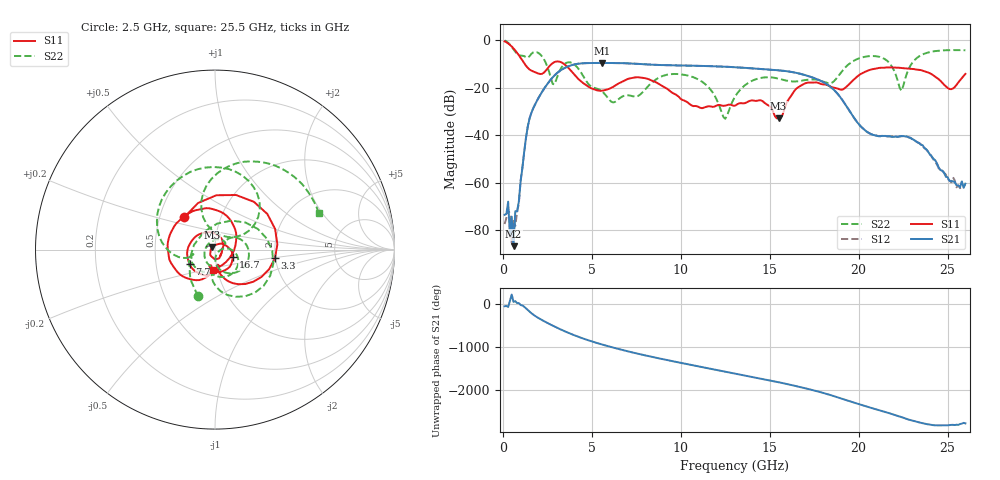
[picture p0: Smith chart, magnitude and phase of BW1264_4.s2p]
!Keysight Technologies,N5245B,MY57181159,A.13.60.06
!Date: Friday, December 18, 2020 23:52:07
!Correction: S11(Full 2 Port(1,2))
!S21(Full 2 Port(1,2))
!S12(Full 2 Port(1,2))
!S22(Full 2 Port(1,2))
!S2P File: Measurements: S11, S21, S12, S22:
# Hz S  dB  R 50
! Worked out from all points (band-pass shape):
!   260 points, 100 MHz to 26 GHz, reference 50 ohm
!   highest |S21| = -9.65 dB at 5.6 GHz (marker M1); lowest = -86.7 dB at 600 MHz (marker M2)
!   |S21| within 3 dB of the highest: 3.273 GHz to 15.35 GHz (12.08 GHz wide, 130 % of centre)
!   lowest |S11| = -33.0 dB at 15.5 GHz (marker M3), VSWR 1.05, Z = 48.3 + j1.35 ohm
!   |S11| at or under -10 dB: 1.223 GHz to 2.759 GHz (1.535 GHz wide, 77.1 % of centre); 3.421 GHz to end of sweep
!   |S22| runs from -33.1 to -0.2 dB; largest |S21 - S12| = 0.00052
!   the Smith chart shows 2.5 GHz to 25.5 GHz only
!   S11 on the Smith chart (normalised r, x): 2.5 GHz: 0.67, +0.26; 3.3 GHz: 1.99, -0.22; 7.7 GHz: 0.74, -0.13; 16.7 GHz: 1.22, -0.10; 25.5 GHz: 0.95, -0.22
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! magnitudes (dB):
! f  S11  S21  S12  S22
! 100 MHz  -0.6  -73.5  -77.4  -0.2
! 300 MHz  -1.5  -68.0  -71.5  -1.2
! 400 MHz  -2.1  -82.7  -73.0  -1.9
! 600 MHz  -3.5  -86.7  -75.3  -3.9
! 1.5 GHz  -12.4  -33.1  -33.0  -6.8
! 2.5 GHz  -12.1  -18.5  -18.5  -11.2
! 3.3 GHz  -9.4  -12.5  -12.5  -11.5
! 4.5 GHz  -18.0  -9.8  -9.8  -14.9
! 5.6 GHz  -21.3  -9.6  -9.6  -21.7
! 7.7 GHz  -15.7  -10.1  -10.1  -23.1
! 8.8 GHz  -18.6  -10.5  -10.5  -15.7
! 11.2 GHz  -28.7  -10.9  -10.9  -17.6
! 12.5 GHz  -27.6  -11.2  -11.2  -33.1
! 13.1 GHz  -27.4  -11.5  -11.5  -23.2
! 15.5 GHz  -33.0  -12.7  -12.7  -16.3
! 16.7 GHz  -19.4  -14.2  -14.2  -17.2
! 17.4 GHz  -17.9  -15.7  -15.7  -16.6
! 21.7 GHz  -11.5  -40.4  -40.6  -9.5
! 22.4 GHz  -11.8  -40.4  -40.5  -21.3
! 23.3 GHz  -12.5  -43.0  -43.0  -7.4
! 25.5 GHz  -18.9  -61.1  -62.0  -4.3
! 26 GHz  -14.3  -60.4  -61.0  -4.3
